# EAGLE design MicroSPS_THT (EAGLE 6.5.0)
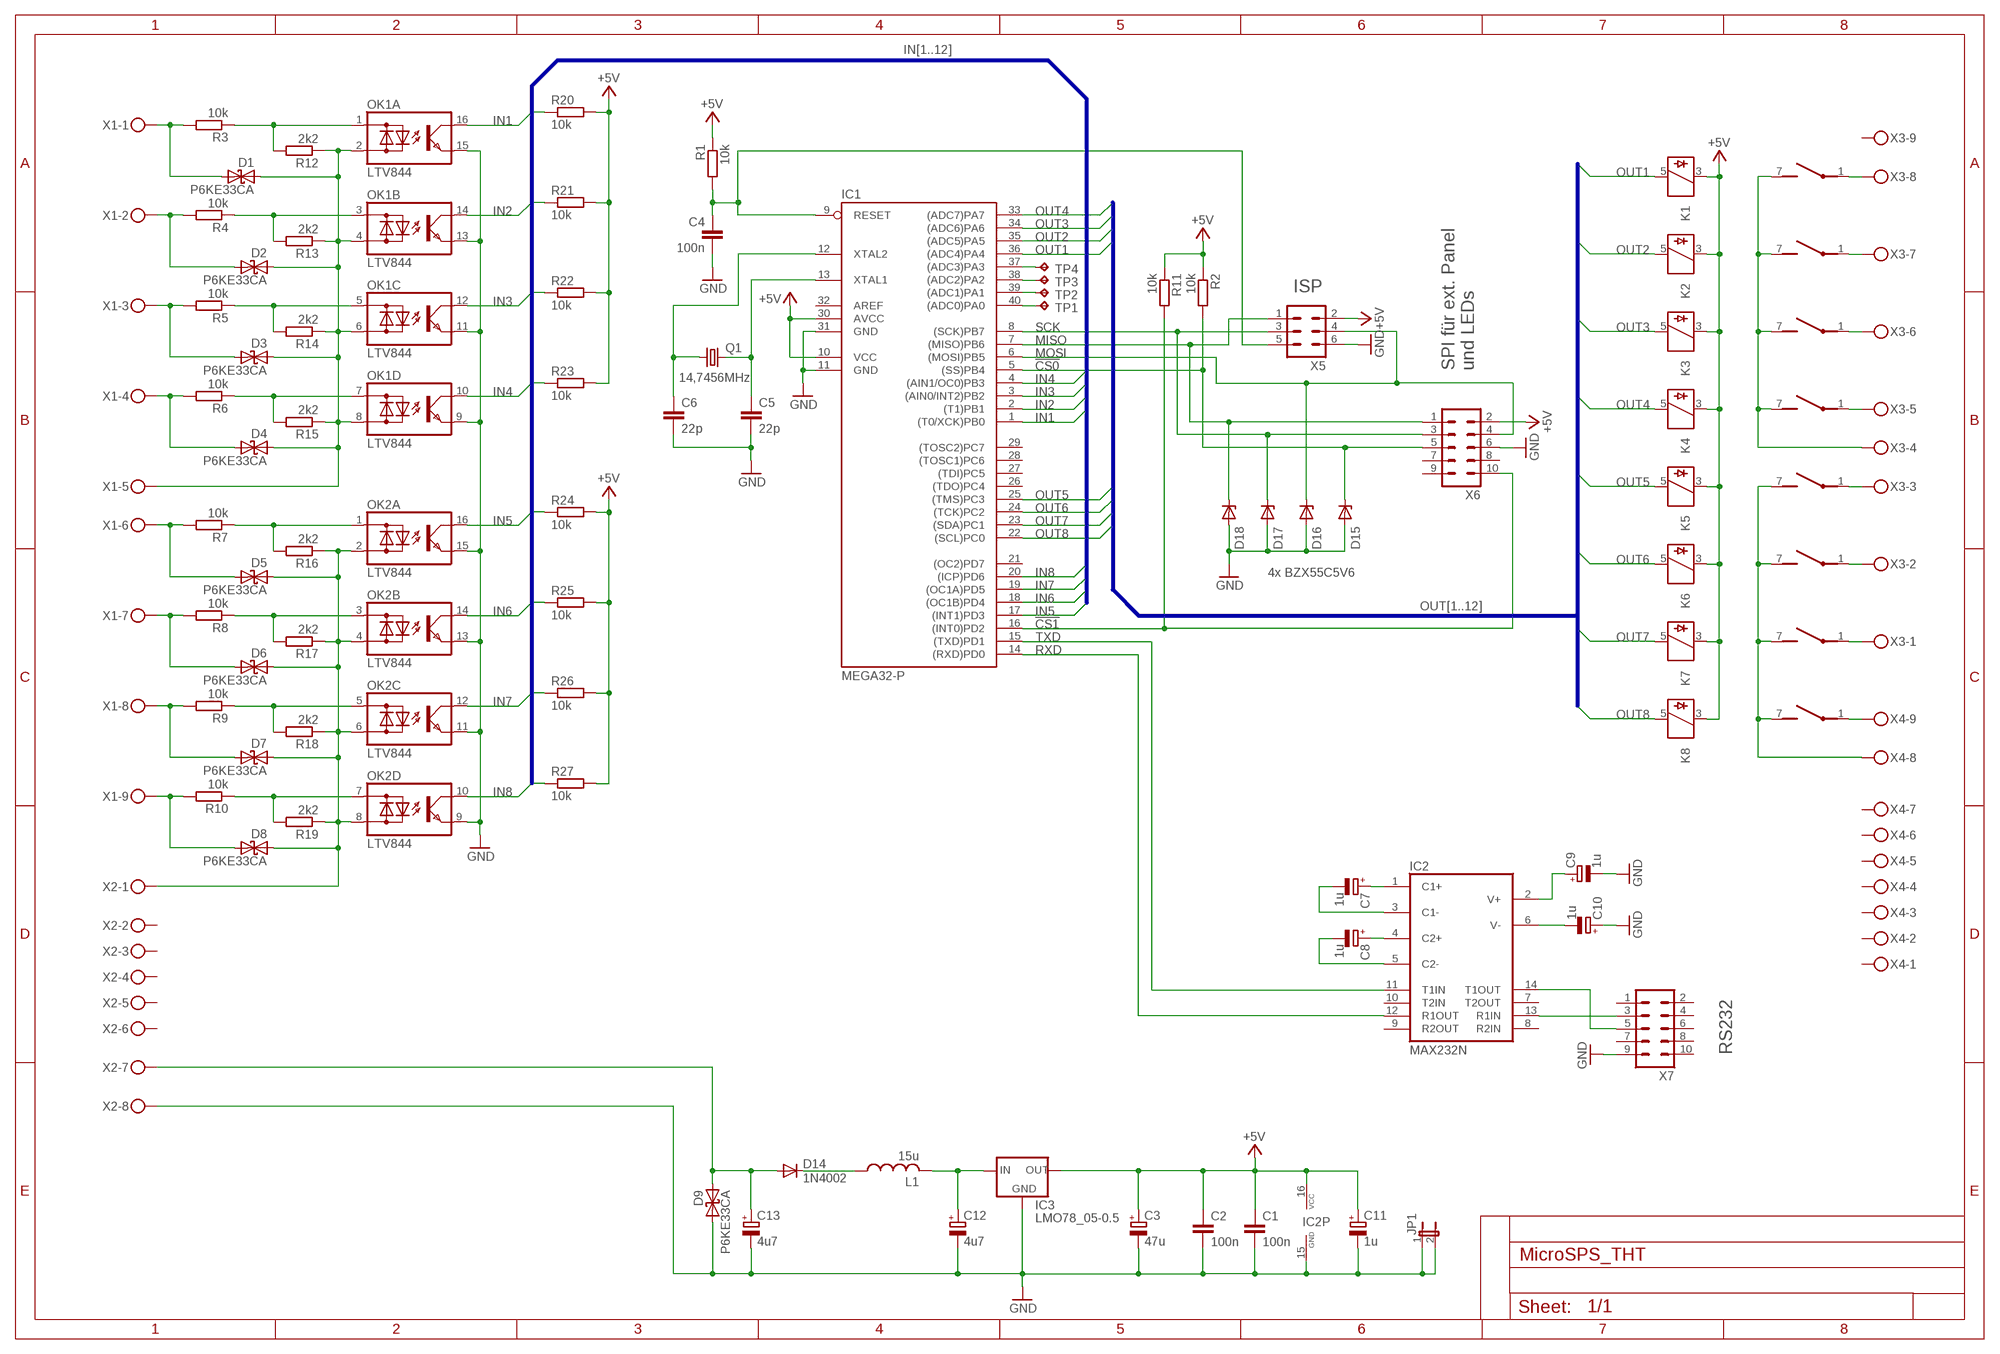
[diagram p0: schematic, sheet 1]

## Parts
C1  100n  C-EU025-024X044  [C025-024X044]
C2  100n  C-EU025-024X044  [C025-024X044]
C3  47u  CPOL-EUE2.5-5  [E2,5-5]
C4  100n  C-EU025-024X044  [C025-024X044]
C5  22p  C-EU025-024X044  [C025-024X044]
C6  22p  C-EU025-024X044  [C025-024X044]
C7  1u  CPOL-EUE2-4  [E2-4]
C8  1u  CPOL-EUE2-4  [E2-4]
C9  1u  CPOL-EUE2-4  [E2-4]
C10  1u  CPOL-EUE2-4  [E2-4]
C11  1u  CPOL-EUE2-4  [E2-4]
C12  4u7  CPOL-EUE2-5  [E2-5]
C13  4u7  CPOL-EUE2-5  [E2-5]
D1  P6KE33CA  SUPPRESSOR_BI-DO41  [D-5-BI]
D2  P6KE33CA  SUPPRESSOR_BI-DO41  [D-5-BI]
D3  P6KE33CA  SUPPRESSOR_BI-DO41  [D-5-BI]
D4  P6KE33CA  SUPPRESSOR_BI-DO41  [D-5-BI]
D5  P6KE33CA  SUPPRESSOR_BI-DO41  [D-5-BI]
D6  P6KE33CA  SUPPRESSOR_BI-DO41  [D-5-BI]
D7  P6KE33CA  SUPPRESSOR_BI-DO41  [D-5-BI]
D8  P6KE33CA  SUPPRESSOR_BI-DO41  [D-5-BI]
D9  P6KE33CA  SUPPRESSOR_BI-DO41  [D-5-BI]
D14  1N4002  DIODE-D-2.5  [D-2.5]
D15  ZENER-DIODEZD-7.5  [ZDIO-7.5]
D16  ZENER-DIODEZD-7.5  [ZDIO-7.5]
D17  ZENER-DIODEZD-7.5  [ZDIO-7.5]
D18  ZENER-DIODEZD-7.5  [ZDIO-7.5]
IC1  MEGA32-P  [DIL40]
IC2  MAX232N  MAX232  [DIL16]
IC3  LMO78_05-0.5  78XXS  [78XXS]
JP1  JP1E  [JP1]
K1  35701331  [REED]
K2  35701331  [REED]
K3  35701331  [REED]
K4  35701331  [REED]
K5  35701331  [REED]
K6  35701331  [REED]
K7  35701331  [REED]
K8  35701331  [REED]
L1  15u  L-US0207/2V  [0207/2V]
OK1  LTV844  ILQ620  [DIL16]
OK2  LTV844  ILQ620  [DIL16]
Q1  14,7456MHz  CRYSTALHC49S  [HC49/S]
R1  10k  R-EU_0207/2V  [0207/2V]
R2  10k  R-EU_0207/2V  [0207/2V]
R3  10k  R-EU_0207/2V  [0207/2V]
R4  10k  R-EU_0207/2V  [0207/2V]
R5  10k  R-EU_0207/2V  [0207/2V]
R6  10k  R-EU_0207/2V  [0207/2V]
R7  10k  R-EU_0207/2V  [0207/2V]
R8  10k  R-EU_0207/2V  [0207/2V]
R9  10k  R-EU_0207/2V  [0207/2V]
R10  10k  R-EU_0207/2V  [0207/2V]
R11  10k  R-EU_0207/2V  [0207/2V]
R12  2k2  R-EU_0207/2V  [0207/2V]
R13  2k2  R-EU_0207/2V  [0207/2V]
R14  2k2  R-EU_0207/2V  [0207/2V]
R15  2k2  R-EU_0207/2V  [0207/2V]
R16  2k2  R-EU_0207/2V  [0207/2V]
R17  2k2  R-EU_0207/2V  [0207/2V]
R18  2k2  R-EU_0207/2V  [0207/2V]
R19  2k2  R-EU_0207/2V  [0207/2V]
R20  10k  R-EU_0207/2V  [0207/2V]
R21  10k  R-EU_0207/2V  [0207/2V]
R22  10k  R-EU_0207/2V  [0207/2V]
R23  10k  R-EU_0207/2V  [0207/2V]
R24  10k  R-EU_0207/2V  [0207/2V]
R25  10k  R-EU_0207/2V  [0207/2V]
R26  10k  R-EU_0207/2V  [0207/2V]
R27  10k  R-EU_0207/2V  [0207/2V]
TP1  TPPAD1-13  [P1-13]
TP2  TPPAD1-13  [P1-13]
TP3  TPPAD1-13  [P1-13]
TP4  TPPAD1-13  [P1-13]
X1  MKDSN1,5/9-5,08  [MKDSN1,5/9-5,08]
X2  MKDSN1,5/8-5,08  [MKDSN1,5/8-5,08]
X3  MKDSN1,5/9-5,08  [MKDSN1,5/9-5,08]
X4  MKDSN1,5/9-5,08  [MKDSN1,5/9-5,08]
X5  ML6  [ML6]
X6  ML10  [ML10]
X7  ML10  [ML10]

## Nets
!CS0: D15.C IC1.5((SS)PB4) R2.2 X6.5
!CS1: IC1.16((INT0)PD2) R11.2 X6.10
+5V: C1.1 C2.1 C3.+ C11.+ IC1.10(VCC) IC1.30(AVCC) IC2.16(VCC) IC3.OUT K1.3 K2.3 K3.3 K4.3 K5.3 K6.3 K7.3 K8.3 R1.1 R2.1 R11.1 R20.2 R21.2 R22.2 R23.2 R24.2 R25.2 R26.2 R27.2 X5.2 X6.2
GND: C1.2 C2.2 C3.- C4.2 C5.2 C6.2 C9.- C10.+ C11.- C12.- C13.- D9.C D15.A D16.A D17.A D18.A IC1.11(GND) IC1.31(GND) IC2.15(GND) IC3.GND JP1.1 JP1.2 OK1.9(D:E) OK1.11(C:E) OK1.13(B:E) OK1.15(A:E) OK2.9(D:E) OK2.11(C:E) OK2.13(B:E) OK2.15(A:E) X2.8 X5.6 X6.6 X7.9
IN1: IC1.1((T0/XCK)PB0) OK1.16(A:C) R20.1
IN2: IC1.2((T1)PB1) OK1.14(B:C) R21.1
IN3: IC1.3((AIN0/INT2)PB2) OK1.12(C:C) R22.1
IN4: IC1.4((AIN1/OC0)PB3) OK1.10(D:C) R23.1
IN5: IC1.17((INT1)PD3) OK2.16(A:C) R24.1
IN6: IC1.18((OC1B)PD4) OK2.14(B:C) R25.1
IN7: IC1.19((OC1A)PD5) OK2.12(C:C) R26.1
IN8: IC1.20((ICP)PD6) OK2.10(D:C) R27.1
MISO: D18.C IC1.7((MISO)PB6) X5.1 X6.1
MOSI: D16.C IC1.6((MOSI)PB5) X5.4 X6.4
N$1: D14.C L1.1
N$2: C6.1 IC1.12(XTAL2) Q1.1
N$3: C7.+ IC2.1(C1+)
N$4: C10.- IC2.6(V-)
N$5: C9.+ IC2.2(V+)
N$6: C5.1 IC1.13(XTAL1) Q1.2
N$7: C8.+ IC2.4(C2+)
N$8: OK1.1(A:AC1) R3.1 R12.2
N$9: OK1.3(B:AC1) R4.1 R13.2
N$10: OK1.5(C:AC1) R5.1 R14.2
N$11: OK1.7(D:AC1) R6.1 R15.2
N$12: D1.A D2.A D3.A D4.A OK1.2(A:AC2) OK1.4(B:AC2) OK1.6(C:AC2) OK1.8(D:AC2) R12.1 R13.1 R14.1 R15.1 X1.5
N$13: D1.C R3.2 X1.1
N$14: D2.C R4.2 X1.2
N$15: D3.C R5.2 X1.3
N$16: D4.C R6.2 X1.4
N$17: OK2.1(A:AC1) R7.1 R16.2
N$18: OK2.3(B:AC1) R8.1 R17.2
N$19: OK2.5(C:AC1) R9.1 R18.2
N$20: OK2.7(D:AC1) R10.1 R19.2
N$21: D5.A D6.A D7.A D8.A OK2.2(A:AC2) OK2.4(B:AC2) OK2.6(C:AC2) OK2.8(D:AC2) R16.1 R17.1 R18.1 R19.1 X2.1
N$22: D5.C R7.2 X1.6
N$23: D6.C R8.2 X1.7
N$24: D7.C R9.2 X1.8
N$25: D8.C R10.2 X1.9
N$26: K1.1(2:P) X3.8
N$27: K2.1(2:P) X3.7
N$28: K3.1(2:P) X3.6
N$29: K4.1(2:P) X3.5
N$30: K1.7(2:S) K2.7(2:S) K3.7(2:S) K4.7(2:S) X3.4
N$31: C7.- IC2.3(C1-)
N$32: K5.1(2:P) X3.3
N$33: K6.1(2:P) X3.2
N$34: K7.1(2:P) X3.1
N$35: K8.1(2:P) X4.9
N$36: K5.7(2:S) K6.7(2:S) K7.7(2:S) K8.7(2:S) X4.8
N$37: C8.- IC2.5(C2-)
N$38: IC1.39((ADC1)PA1) TP2.TP
N$39: IC1.40((ADC0)PA0) TP1.TP
N$40: IC2.13(R1IN) X7.3
N$41: IC2.14(T1OUT) X7.5
N$42: C12.+ IC3.IN L1.2
N$43: C13.+ D9.A D14.A X2.7
N$44: IC1.37((ADC3)PA3) TP4.TP
N$45: IC1.38((ADC2)PA2) TP3.TP
N$57: C4.1 IC1.9(RESET) R1.2 X5.5
OUT1: IC1.36((ADC4)PA4) K1.5
OUT2: IC1.35((ADC5)PA5) K2.5
OUT3: IC1.34((ADC6)PA6) K3.5
OUT4: IC1.33((ADC7)PA7) K4.5
OUT5: IC1.25((TMS)PC3) K5.5
OUT6: IC1.24((TCK)PC2) K6.5
OUT7: IC1.23((SDA)PC1) K7.5
OUT8: IC1.22((SCL)PC0) K8.5
RXD: IC1.14((RXD)PD0) IC2.12(R1OUT)
SCK: D17.C IC1.8((SCK)PB7) X5.3 X6.3
TXD: IC1.15((TXD)PD1) IC2.11(T1IN)
Unconnected: IC1.21((OC2)PD7) IC1.26((TDO)PC4) IC1.27((TDI)PC5) IC1.28((TOSC1)PC6) IC1.29((TOSC2)PC7) IC1.32(AREF) IC2.7(T2OUT) IC2.8(R2IN) IC2.9(R2OUT) IC2.10(T2IN) X2.2 X2.3 X2.4 X2.5 X2.6 X3.9 X4.1 X4.2 X4.3 X4.4 X4.5 X4.6 X4.7 X6.7 X6.8 X6.9 X7.1 X7.2 X7.4 X7.6 X7.7 X7.8 X7.10

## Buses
IN[1..12]
OUT[1..12]

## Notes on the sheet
- ISP
- SPI für ext. Panel
  und LEDs
- 4x BZX55C5V6
- RS232

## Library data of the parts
C1 C2 C4-C6 = rcl:C-EU: CAPACITOR, European symbol
C3 C7-C13 = rcl:CPOL-EU: POLARIZED CAPACITOR, European symbol
D1-D9 = Brunner_KMT:SUPPRESSOR_BI-: Schottky Bidirectional Diode
D14 = diode:DIODE-: DIODE
D15-D18 = diode:ZENER-DIODE: Z-Diode
IC1 = atmel:MEGA32-P: MICROCONTROLLER 32 Kbytes FLASH 2 Kbytes SRAM 1 Kbytes EEPROM USART 8-channel 10 bit ADC Source: www.atmel.com .. doc2503.pdf; MPN: ATMEGA32-16PU; OC_FARNELL: 1661729; OC_NEWARK: 51P1794
IC2 = Brunner:MAX232: RS232 TRANSCEIVER; MF: MAXIM; MPN: MAX232ACPE+; OC_FARNELL: 9723773; OC_NEWARK: 68K4544
IC3 = v-reg:78XXS: VOLTAGE REGULATOR
JP1 = jumper:JP1E: JUMPER
K1-K8 = relay:35701331: RELAY reed, 1 x norm. open with polarity; OC_FARNELL: unknown; OC_NEWARK: unknown
L1 = rcl:L-US: INDUCTOR, American symbol
OK1 OK2 = optocoupler:ILQ620: SIEMENS OPTO COUPLER; MF: VISHAY/TELEFUNKEN; MPN: ILQ620; OC_FARNELL: 1612470; OC_NEWARK: 58K1694
Q1 = crystal:CRYSTAL: CRYSTAL; OC_FARNELL: 1667008; OC_NEWARK: unknown
R1-R27 = rcl:R-EU_: RESISTOR, European symbol
TP1-TP4 = testpad:TP: Test pad
X1 X3 X4 = con-phoenix-508:MKDSN1,5/9-5,08: MKDSN 1,5/ 9-5,08 Printklemme Nennstrom: 13,5 A Nennspannung: 250 V Rastermaß: 5,08 mm Polzahl: 9 Anschlussart: Schraubanschluss Montage: Löten Anschlussrichtung Leiter/Platine: 0 ° Artikelnummer: 1729199 Source: http://eshop.phoenixcontact.com .. 1729199.pdf; MPN: SMKDSN1,5/9-5,08; OC_FARNELL: 1792912; OC_NEWARK: 70R0305
X2 = con-phoenix-508:MKDSN1,5/8-5,08: MKDSN 1,5/ 8-5,08 Printklemme Nennstrom: 13,5 A Nennspannung: 250 V Rastermaß: 5,08 mm Polzahl: 8 Anschlussart: Schraubanschluss Montage: Löten Anschlussrichtung Leiter/Platine: 0 ° Artikelnummer: 1729186 Source: http://eshop.phoenixcontact.com .. 1729186.pdf; MPN: SMKDSN1,5/8-5,08; OC_FARNELL: 1792911; OC_NEWARK: 70R0304
X5 = con-harting-ml:ML6: HARTING; OC_FARNELL: unknown; OC_NEWARK: unknown
X6 X7 = con-ml:ML10: HARTING; OC_FARNELL: unknown; OC_NEWARK: unknown

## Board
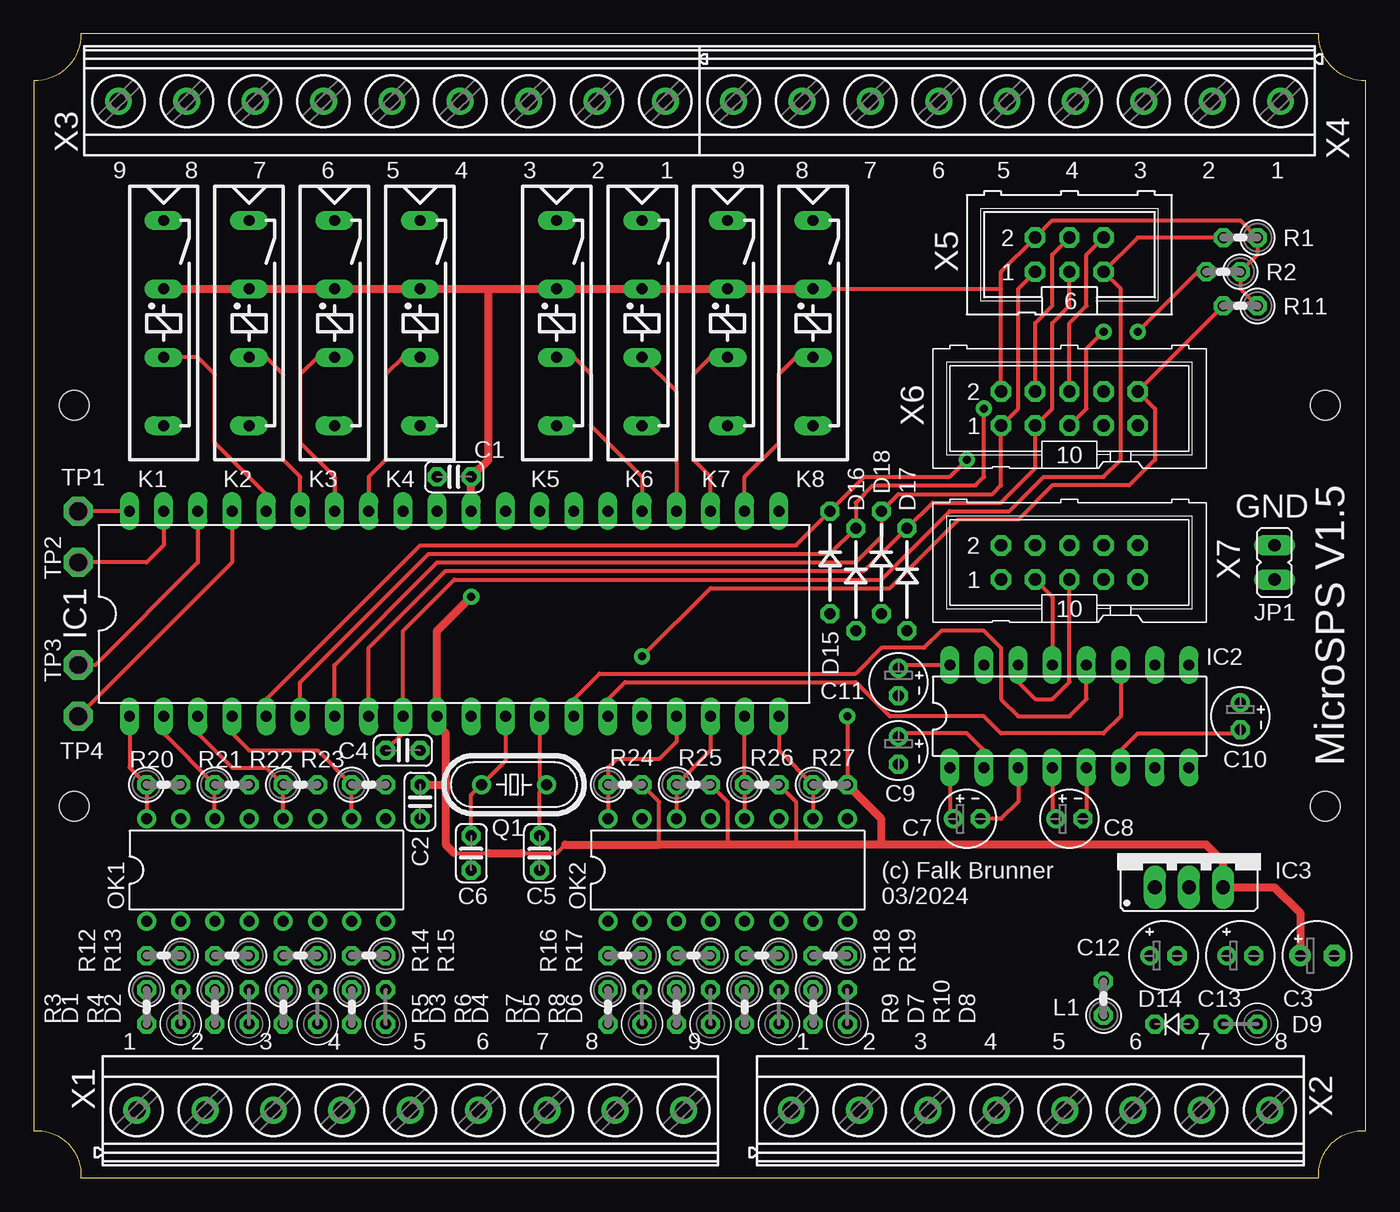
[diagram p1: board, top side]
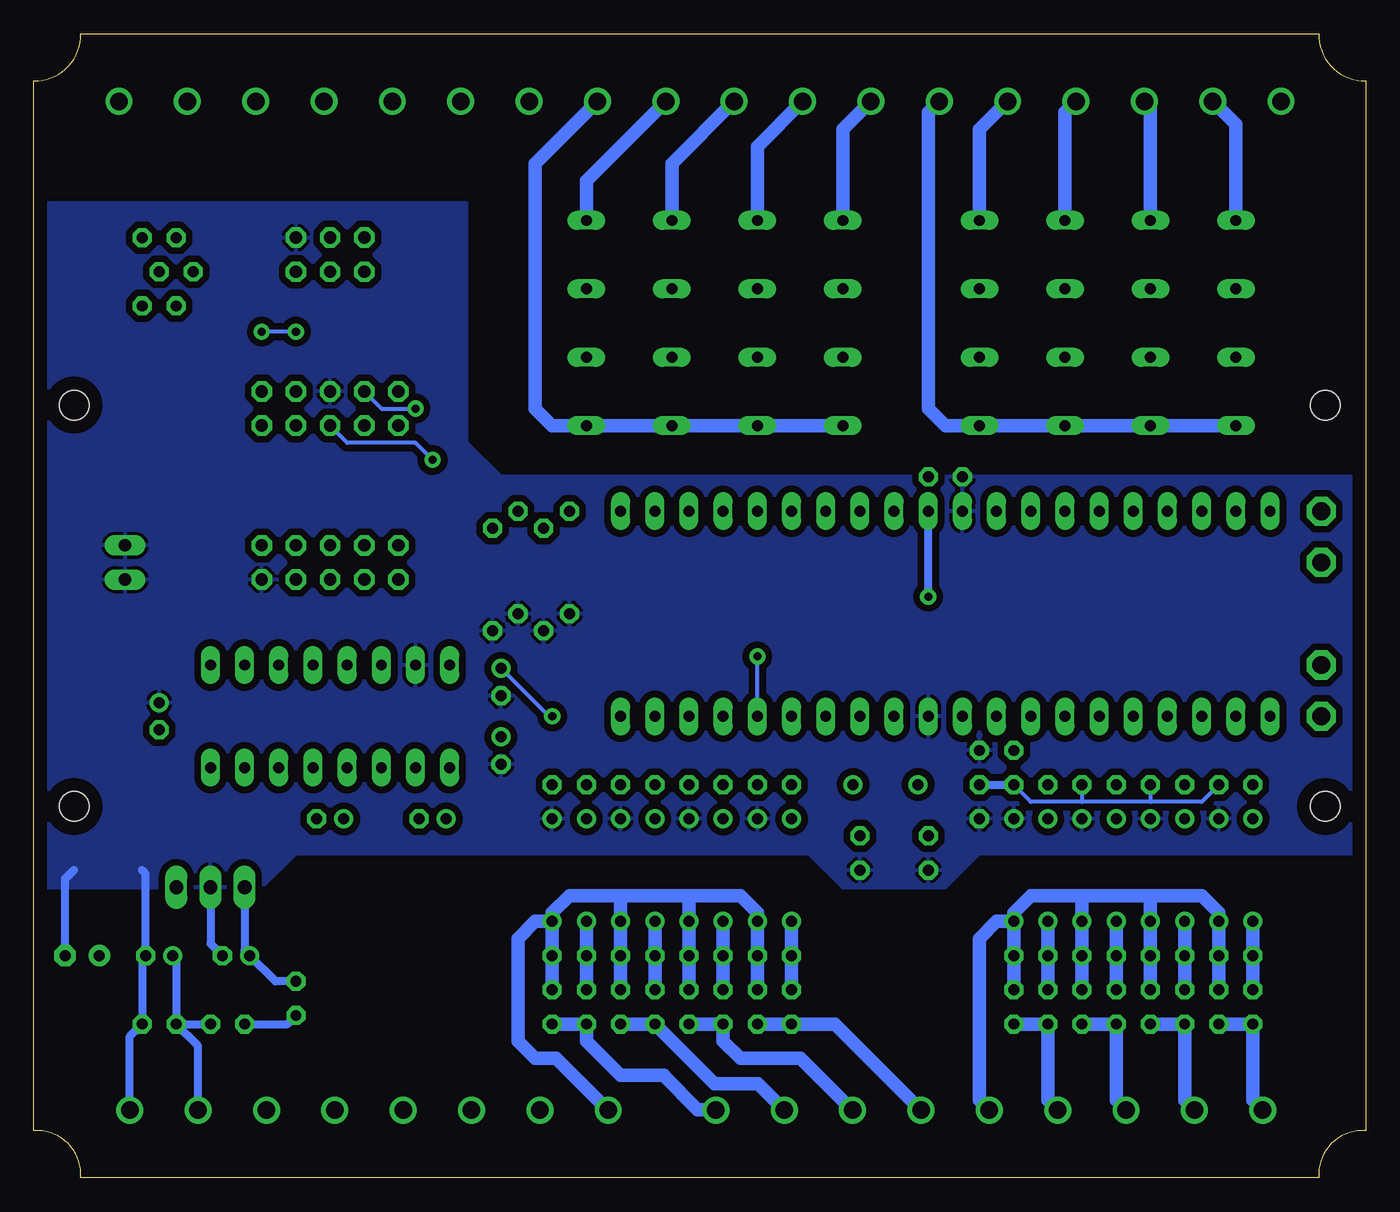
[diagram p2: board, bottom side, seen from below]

Size 99 x 85 mm. Coordinates in mm from the lower left corner, seen from the top.
Outline: 0,3.5 arc-99 3.5,0 95.5,0 arc-99 99,3.5 99,81.5 arc-93 95.5,85 3.5,85 arc-93 0,81.5 0,3.5
Copper layers (1*16): Top 0.035mm / dielectric 1.5mm / Bottom 0.035mm
Design rules "default *": minimum track width 0.3mm, minimum drill 0.6mm, track to track 0.3mm, track to pad 0.3mm, pad to pad 0.3mm, via to via 0.3mm, smd to smd 8mil, copper to edge 1mm, drill to drill 0.3mm, minimum pad ring 0.3mm, minimum via ring 0.3mm, stop-mask expansion 4mil, vias tented up to drill 0mil, thermal gap 10mil
Holes 2.2 mm at 3,57.4 3,27.6 96,57.4 96,27.6

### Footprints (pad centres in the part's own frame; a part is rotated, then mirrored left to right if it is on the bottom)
C025-024X044 = drill 0.813 octagon: 1 -1.27,0; 2 1.27,0
E2,5-5 = drill 0.813 pad 1.6: + -1.27,0 | drill 0.813 pad 1.6 octagon: - 1.27,0
E2-4 = drill 0.813 pad 1.27: + -1.016,0 | drill 0.813 pad 1.27 octagon: - 1.016,0
E2-5 = drill 0.813 pad 1.27: + -1.016,0 | drill 0.813 pad 1.27 octagon: - 1.016,0
D-5-BI = drill 0.813 octagon: A 0,0; C -2.54,0
D-2.5 = drill 0.813 octagon: A 1.27,0; C -1.27,0
ZDIO-7.5 = drill 0.813 octagon: A 3.81,0; C -3.81,0
DIL40 = drill 0.813 long: 1 -24.13,-7.62; 2 -21.59,-7.62; 3 -19.05,-7.62; 4 -16.51,-7.62; 5 -13.97,-7.62; 6 -11.43,-7.62; 7 -8.89,-7.62; 8 -6.35,-7.62; 9 -3.81,-7.62; 10 -1.27,-7.62; 11 1.27,-7.62; 12 3.81,-7.62; 13 6.35,-7.62; 14 8.89,-7.62; 15 11.43,-7.62; 16 13.97,-7.62; 17 16.51,-7.62; 18 19.05,-7.62; 19 21.59,-7.62; 20 24.13,-7.62; 21 24.13,7.62; 22 21.59,7.62; 23 19.05,7.62; 24 16.51,7.62; 25 13.97,7.62; 26 11.43,7.62; 27 8.89,7.62; 28 6.35,7.62; 29 3.81,7.62; 30 1.27,7.62; 31 -1.27,7.62; 32 -3.81,7.62; 33 -6.35,7.62; 34 -8.89,7.62; 35 -11.43,7.62; 36 -13.97,7.62; 37 -16.51,7.62; 38 -19.05,7.62; 39 -21.59,7.62; 40 -24.13,7.62
DIL16 = drill 0.813 long: 1 -8.89,-3.81; 2 -6.35,-3.81; 3 -3.81,-3.81; 4 -1.27,-3.81; 5 1.27,-3.81; 6 3.81,-3.81; 7 6.35,-3.81; 8 8.89,-3.81; 9 8.89,3.81; 10 6.35,3.81; 11 3.81,3.81; 12 1.27,3.81; 13 -1.27,3.81; 14 -3.81,3.81; 15 -6.35,3.81; 16 -8.89,3.81
78XXS = drill 1.016 long: GND 0,-2.54; IN -2.54,-2.54; OUT 2.54,-2.54
JP1 = drill 0.914 long: 1 0,-1.27; 2 0,1.27
REED = drill 0.813 long: 1 -17.78,2.54; 3 -12.7,2.54; 5 -7.62,2.54; 7 -2.54,2.54
0207/2V = drill 0.813 octagon: 1 -1.27,0; 2 1.27,0
DIL16' = drill 0.813: 1 -8.89,-3.81; 2 -6.35,-3.81; 3 -3.81,-3.81; 4 -1.27,-3.81; 5 1.27,-3.81; 6 3.81,-3.81; 7 6.35,-3.81; 8 8.89,-3.81; 9 8.89,3.81; 10 6.35,3.81; 11 3.81,3.81; 12 1.27,3.81; 13 -1.27,3.81; 14 -3.81,3.81; 15 -6.35,3.81; 16 -8.89,3.81
HC49/S = drill 0.813: 1 -2.413,0; 2 2.413,0
P1-13 = drill 1.321 pad 2.159 octagon: TP 0,0
MKDSN1,5/9-5,08 = drill 1.3 pad 2: 1 -20.341,0.025; 2 -15.261,0.025; 3 -10.181,0.025; 4 -5.101,0.025; 5 -0.021,0.025; 6 5.059,0.025; 7 10.139,0.025; 8 15.219,0.025; 9 20.299,0.025
MKDSN1,5/8-5,08 = drill 1.3 pad 2: 1 -17.801,0.025; 2 -12.721,0.025; 3 -7.641,0.025; 4 -2.561,0.025; 5 2.519,0.025; 6 7.599,0.025; 7 12.679,0.025; 8 17.759,0.025
ML6 = drill 0.914 octagon: 1 -2.54,-1.27; 2 -2.54,1.27; 3 0,-1.27; 4 0,1.27; 5 2.54,-1.27; 6 2.54,1.27
ML10 = drill 0.914 octagon: 1 -5.08,-1.27; 2 -5.08,1.27; 3 -2.54,-1.27; 4 -2.54,1.27; 5 0,-1.27; 6 0,1.27; 7 2.54,-1.27; 8 2.54,1.27; 9 5.08,-1.27; 10 5.08,1.27

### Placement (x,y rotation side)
C1  31.25,52.07 180 top
C2  28.71,27.94 270 top
C3  95.39,16.51 0 top
C4  27.44,31.75 0 top
C5  37.6,24.13 270 top
C6  32.52,24.13 270 top
C7  69.35,26.67 0 top
C8  76.97,26.67 0 top
C9  64.27,31.75 270 top
C10  89.67,34.29 270 top
C11  64.27,36.83 270 top
C12  83.95,16.51 0 top
C13  89.67,16.51 0 top
D1  10.93,13.97 90 top
D2  16.01,13.97 90 top
D3  21.09,13.97 90 top
D4  26.17,13.97 90 top
D5  45.22,13.97 90 top
D6  50.3,13.97 90 top
D7  55.38,13.97 90 top
D8  60.46,13.97 90 top
D9  88.4,11.43 180 top
D14  84.59,11.43 0 top
D15  59.19,45.72 270 top
D16  61.09,44.45 270 top
D17  64.91,44.45 270 top
D18  63,45.72 270 top
IC1  31.25,41.91 0 top
IC2  76.97,34.29 0 top
IC3  85.86,24.13 0 top
JP1  92.21,45.72 180 top
K1  7.12,53.34 270 top
K2  13.47,53.34 270 top
K3  19.82,53.34 270 top
K4  26.17,53.34 270 top
K5  36.33,53.34 270 top
K6  42.68,53.34 270 top
K7  49.03,53.34 270 top
K8  55.38,53.34 270 top
L1  79.51,13.34 90 top
OK1  LTV844  [DIL16']  17.28,22.86 0 top
OK2  LTV844  [DIL16']  51.57,22.86 0 top
Q1  35.7,29.21 0 top
R1  89.67,69.85 180 top
R2  88.4,67.31 180 top
R3  8.39,12.7 270 top
R4  13.47,12.7 270 top
R5  18.55,12.7 270 top
R6  23.63,12.7 270 top
R7  42.68,12.7 270 top
R8  47.76,12.7 270 top
R9  52.84,12.7 270 top
R10  57.92,12.7 270 top
R11  89.67,64.77 180 top
R12  9.66,16.51 180 top
R13  14.74,16.51 180 top
R14  19.82,16.51 180 top
R15  24.9,16.51 180 top
R16  43.95,16.51 180 top
R17  49.03,16.51 180 top
R18  54.11,16.51 180 top
R19  59.19,16.51 180 top
R20  9.66,29.21 0 top
R21  14.74,29.21 0 top
R22  19.82,29.21 0 top
R23  24.9,29.21 0 top
R24  43.95,29.21 0 top
R25  49.03,29.21 0 top
R26  54.11,29.21 0 top
R27  59.19,29.21 0 top
TP1  3.31,49.53 0 top
TP2  3.31,45.72 0 top
TP3  3.31,38.1 0 top
TP4  3.31,34.29 0 top
U$1  [A4L-LOC]  not placed on the board
X1  28,5 0 top
X2  74.1,5 0 top
X3  26.6,80 180 top
X4  72.32,80 180 top
X5  76.97,68.58 0 top
X6  76.97,57.15 0 top
X7  76.97,45.72 0 top

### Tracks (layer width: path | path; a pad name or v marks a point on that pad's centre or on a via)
!CS0  (via drill 0.6)
  Top 0.305: IC1.5 17.28,35.56 28.71,46.99 56.65,46.99 D15.C 61.73,52.07 68.08,52.07 v69.35,53.34 | X6.5 78.24,57.15 78.24,61.59 v79.51,62.87 | R2.2 86.5,67.31 v82.05,62.87
  Bottom 0.305: v69.35,53.34 70.62,54.61 75.7,54.61 X6.5 | v79.51,62.87 v82.05,62.87
!CS1  (via drill 0.6)
  Top 0.305: v45.22,38.73 50.3,43.81 63.64,43.81 68.72,48.9 73.16,48.9 75.7,51.44 81.42,51.44 83.32,53.34 83.32,57.15 X6.10 R11.2
  Bottom 0.305: IC1.16 v45.22,38.73
+5V  (via drill 0.6)
  Top 0.305: 46.49,24.77 46.49,27.94 R24.2 | X6.2 71.89,66.04 | 71.89,66.04 71.89,67.31 X5.2 75.7,71.12 89.67,71.12 R1.1 90.94,68.58 R2.1 89.67,66.04 R11.1 | K8.3 71.89,66.04 | R25.2 51.57,27.94 51.57,24.77 | R26.2 56.65,27.94 56.65,24.77 | 39.51,24.77 38.87,24.13 36.33,24.13 | v60.46,34.29 R27.2 | 31.25,24.13 33.79,24.13 | IC2.16 64.52,38.1 C11.+
  Top 0.61: 31.25,24.13 30.61,24.77 30.61,29.21 | K1.3 K2.3 K3.3 K4.3 33.79,66.04 | 33.79,66.04 K5.3 K6.3 K7.3 K8.3 | IC1.30 C1.1 33.79,53.34 33.79,66.04 | 63,24.77 87.13,24.77 88.4,23.5 IC3.OUT 92.21,21.59 94.11,19.68 C3.+ | 63,24.77 63,26.67 R27.2 | 63,24.77 56.65,24.77 51.57,24.77 46.49,24.77 39.51,24.77 | 30.61,29.21 30.61,33.02 29.98,33.66 IC1.10 29.98,40.64 v32.52,43.18 | C2.1 30.61,29.21 | 33.79,24.13 36.33,24.13
  Bottom 0.305: R20.2 12.2,27.94 16.01,27.94 | 16.01,27.94 21.09,27.94 | 21.09,27.94 24.9,27.94 R23.2 | R21.2 16.01,27.94 | R22.2 21.09,27.94 | v60.46,34.29 60.71,34.29 C11.+
  Bottom 0.61: C2.1 R23.2 | v32.52,43.18 IC1.30
GND
  Top 0.305: X6.6 76.97,63.5 78.24,64.77 78.24,68.58 X5.6
  Bottom 0.61: X2.8 91.86,10.51 D9.C 90.94,16.26 C13.- 90.69,22.61 90.94,22.86 | IC3.GND 85.86,17.4 C12.- | C3.- 96.66,22.23 96.02,22.86
  pour Bottom (isolate 0.5): -1.77,52.07 64.27,52.07 66.81,54.61 66.81,72.39 99.83,72.39 99.83,21.59 82.05,21.59 79.51,24.13 41.41,24.13 38.87,21.59 31.25,21.59 28.71,24.13 -1.77,24.13
IN1
  Top 0.305: OK1.16 R20.1 7.12,30.48 IC1.1
IN2
  Top 0.305: OK1.14 R21.1 9.66,33.02 IC1.2
IN3
  Top 0.305: OK1.12 R22.1 17.28,30.48 14.74,30.48 12.2,33.02 IC1.3
IN4
  Top 0.305: OK1.10 R23.1 21.09,31.75 16.01,31.75 14.74,33.02 IC1.4
IN5
  Top 0.305: OK2.16 R24.1 42.68,30.48 43.31,31.11 46.49,31.11 47.76,32.38 IC1.17
IN6
  Top 0.305: OK2.14 R25.1 50.3,31.75 IC1.18
IN7
  Top 0.305: OK2.12 R26.1 IC1.19
IN8
  Top 0.305: IC1.20 55.38,31.75 R27.1 OK2.10
MISO
  Top 0.305: IC1.7 22.36,38.1 29.98,45.72 61.09,45.72 63,47.62 D18.C 64.27,50.8 71.25,50.8 71.89,51.44 X6.1 73.16,57.15 73.16,66.04 X5.1
MOSI  (via drill 0.6)
  Top 0.305: IC1.6 19.82,36.83 29.34,46.35 59.19,46.35 D16.C 61.09,50.16 62.37,51.44 69.98,51.44 70.62,52.07 v70.62,57.15 | X6.4 74.43,63.5 75.7,64.77 75.7,68.58 X5.4
  Bottom 0.305: X6.4 73.16,57.15 v70.62,57.15
N$1
  Bottom 0.61: D14.C 80.14,11.43 L1.1
N$2
  Top 0.305: IC1.12 35.06,30.99 Q1.1 32.52,28.45 C6.1
N$3
  Top 0.305: IC2.1 68.08,26.92 C7.+
N$4
  Top 0.305: IC2.6 80.78,31.75 82.05,33.02 89.42,33.02 C10.-
N$5
  Top 0.305: IC2.2 70.62,31.75 69.35,33.02 64.52,33.02 C9.+
N$6
  Top 0.305: IC1.13 37.6,29.72 Q1.2 37.6,28.7 C5.1
N$7
  Top 0.305: IC2.4 75.7,26.92 C8.+
N$8
  Bottom 1.016: OK1.1 R12.2 R3.1
N$9
  Bottom 1.016: OK1.3 R13.2 R4.1
N$10
  Bottom 1.016: OK1.5 R14.2 R5.1
N$11
  Bottom 1.016: OK1.7 R15.2 R6.1
N$12
  Bottom 1.016: D1.A R12.1 OK1.2 10.93,19.68 12.2,20.95 12.84,20.95 16.01,20.95 | 16.01,20.95 21.09,20.95 | 21.09,20.95 24.27,20.95 24.9,20.95 26.17,19.68 OK1.8 | X1.5 28.71,5.76 28.71,16.51 28.71,17.78 27.44,19.05 OK1.8 | 21.09,20.95 OK1.6 R14.1 D3.A | 16.01,20.95 OK1.4 R13.1 D2.A | OK1.8 R15.1 D4.A
N$13
  Bottom 1.016: X1.1 8.39,5.76 R3.2 D1.C
N$14
  Bottom 1.016: X1.2 13.47,5.76 R4.2 D2.C
N$15
  Bottom 1.016: X1.3 18.55,5.76 R5.2 D3.C
N$16
  Bottom 1.016: X1.4 23.63,5.76 R6.2 D4.C
N$17
  Bottom 1.016: OK2.1 R16.2 R7.1
N$18
  Bottom 1.016: OK2.3 R17.2 R8.1
N$19
  Bottom 1.016: OK2.5 R18.2 R9.1
N$20
  Bottom 1.016: OK2.7 R19.2 R10.1
N$21
  Bottom 1.016: D5.A R16.1 OK2.2 45.22,19.68 46.49,20.95 50.3,20.95 | 50.3,20.95 55.38,20.95 | 55.38,20.95 59.19,20.95 60.46,19.68 OK2.8 | D6.A R17.1 OK2.4 50.3,20.95 | D7.A R18.1 OK2.6 55.38,20.95 | D8.A R19.1 OK2.8 | OK2.8 61.73,19.05 63,17.78 63,10.16 61.73,8.89 60.16,8.89 X2.1
N$22
  Bottom 1.016: D5.C R7.2 39.46,11.43 X1.6
N$23
  Bottom 1.016: D6.C R8.2 47.76,10.16 46.49,8.89 42,8.89 X1.7
N$24
  Bottom 1.016: D7.C R9.2 48.4,6.99 45.18,6.99 X1.8
N$25
  Bottom 1.016: D8.C R10.2 57.92,10.16 55.38,7.62 52.16,7.62 52.16,7.58 49.66,5.08 48.35,5.08 X1.9
N$26
  Bottom 1.016: K1.1 9.66,78.25 X3.8
N$27
  Bottom 1.016: K2.1 16.01,79.52 X3.7
N$28
  Bottom 1.016: K3.1 22.36,79.16 X3.6
N$29
  Bottom 1.016: K4.1 28.71,77.89 X3.5
N$30
  Bottom 1.016: K1.7 K2.7 K3.7 K4.7 31.25,55.88 32.52,57.15 32.52,79.16 X3.4
N$31
  Top 0.305: IC2.3 73.16,27.94 71.89,26.67 C7.-
N$32
  Bottom 1.016: K5.1 38.87,77.89 X3.3
N$33
  Bottom 1.016: K6.1 45.22,76.62 X3.2
N$34
  Bottom 1.016: K7.1 51.57,75.35 X3.1
N$35
  Bottom 1.016: K8.1 57.92,74.08 X4.9
N$36
  Bottom 1.016: K5.7 K6.7 K7.7 K8.7 60.46,55.88 61.73,57.15 61.73,75.35 X4.8
N$37
  Top 0.305: IC2.5 78.24,26.92 C8.-
N$38
  Top 0.305: IC1.39 9.66,46.99 8.39,45.72 TP2.TP
N$39
  Top 0.305: IC1.40 TP1.TP
N$40
  Top 0.305: X7.3 75.7,43.18 IC2.13
N$41
  Top 0.305: IC2.14 73.16,36.83 74.43,35.56 75.7,35.56 76.97,36.83 X7.5
N$42
  Bottom 0.61: IC3.IN 83.32,16.89 C12.+ 81.03,14.61 L1.2
N$43
  Bottom 0.61: C13.+ 88.4,16.26 D9.A | D9.A D14.A | X2.7 86.78,9.81 D9.A
N$44
  Top 0.305: IC1.37 14.74,45.72 TP4.TP
N$45
  Top 0.305: IC1.38 12.2,45.72 4.58,38.1 TP3.TP
N$57
  Top 0.305: C4.1 27.44,33.02 IC1.9 27.44,40.64 31.25,44.45 63,44.45 68.08,49.53 72.53,49.53 75.06,52.07 79.51,52.07 80.78,53.34 80.78,66.04 X5.5 82.05,69.85 R1.2
OUT1
  Top 0.305: IC1.36 17.28,50.8 13.47,54.61 13.47,59.69 12.2,60.96 K1.5
OUT2
  Top 0.305: IC1.35 19.82,52.07 18.55,53.34 18.55,59.69 17.28,60.96 K2.5
OUT3
  Top 0.305: K3.5 21.09,60.96 19.82,59.69 19.82,54.61 22.36,52.07 IC1.34
OUT4
  Top 0.305: K4.5 27.44,60.96 26.17,59.69 26.17,53.34 24.9,52.07 IC1.33
OUT5
  Top 0.305: K5.5 40.14,60.96 41.41,59.69 41.41,55.88 45.22,52.07 IC1.25
OUT6
  Top 0.305: K6.5 47.76,58.42 IC1.24
OUT7
  Top 0.305: IC1.23 50.3,52.07 49.03,53.34 49.03,59.69 50.3,60.96 K7.5
OUT8
  Top 0.305: IC1.22 52.84,52.07 55.38,54.61 55.38,59.69 56.65,60.96 K8.5
RXD
  Top 0.305: IC1.14 40.14,35.56 42.05,37.47 61.09,37.47 63,39.37 66.17,39.37 67.44,40.64 70.62,40.64 71.89,39.37 71.89,35.56 73.16,34.29 76.97,34.29 78.24,35.56 IC2.12
SCK
  Top 0.305: IC1.8 24.9,39.37 30.61,45.09 61.73,45.09 D17.C 66.81,50.16 71.89,50.16 74.43,52.7 X6.3 75.7,57.15 75.7,63.5 76.97,64.77 X5.3
TXD
  Top 0.305: IC1.15 42.68,35.56 43.95,36.83 61.09,36.83 63.64,34.29 70.62,34.29 71.89,33.02 79.51,33.02 80.78,34.29 IC2.11

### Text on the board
tPlace: 9 | 8 | 7 | 6 | 5 | 4 | 3 | 2 | 1 | 9 | 8 | 7 | 6 | 5 | 4 | 3 | 2 | 1 | GND | MicroSPS V1.5 | (c) Falk Brunner / 03/2024 | 1 | 2 | 3 | 4 | 5 | 6 | 7 | 8 | 9 | 1 | 2 | 3 | 4 | 5 | 6 | 7 | 8
_tPlace: 9 | 8 | 7 | 6 | 5 | 4 | 3 | 2 | 1 | 9 | 8 | 7 | 6 | 5 | 4 | 3 | 2 | 1 | MicroSPS V1.1 | GND | (c) Falk Brunner 09/2020 | 1 | 2 | 3 | 4 | 5 | 6 | 7 | 8 | 9 | 1 | 2 | 3 | 4 | 5 | 6 | 7 | 8
_tNames: X4 | X3 | X5 | K1 | K2 | K3 | K4 | K5 | K6 | K7 | K8 | K9 | K10 | K11 | K12 | TP1 | Q1 | C5 | C11 | R11 | JP1 | X7 | X6 | C1 | IC2 | C2 | C6 | C9 | C4 | R1 | IC1 | C7 | C8 | C10 | D17 | R2 | D18 | D15 | D16 | R20 | R21 | R22 | R23 | R24 | R25 | R26 | R27 | R36 | R37 | R38 | R39 | C3 | IC3 | OK1 | OK2 | OK3 | C12 | C13 | D13 | L1 | D14 | X2 | X1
